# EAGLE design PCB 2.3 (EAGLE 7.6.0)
CNAME: DIY-Thermocam V2; CREVISION: 2.3; DESIGNER: Max Ritter
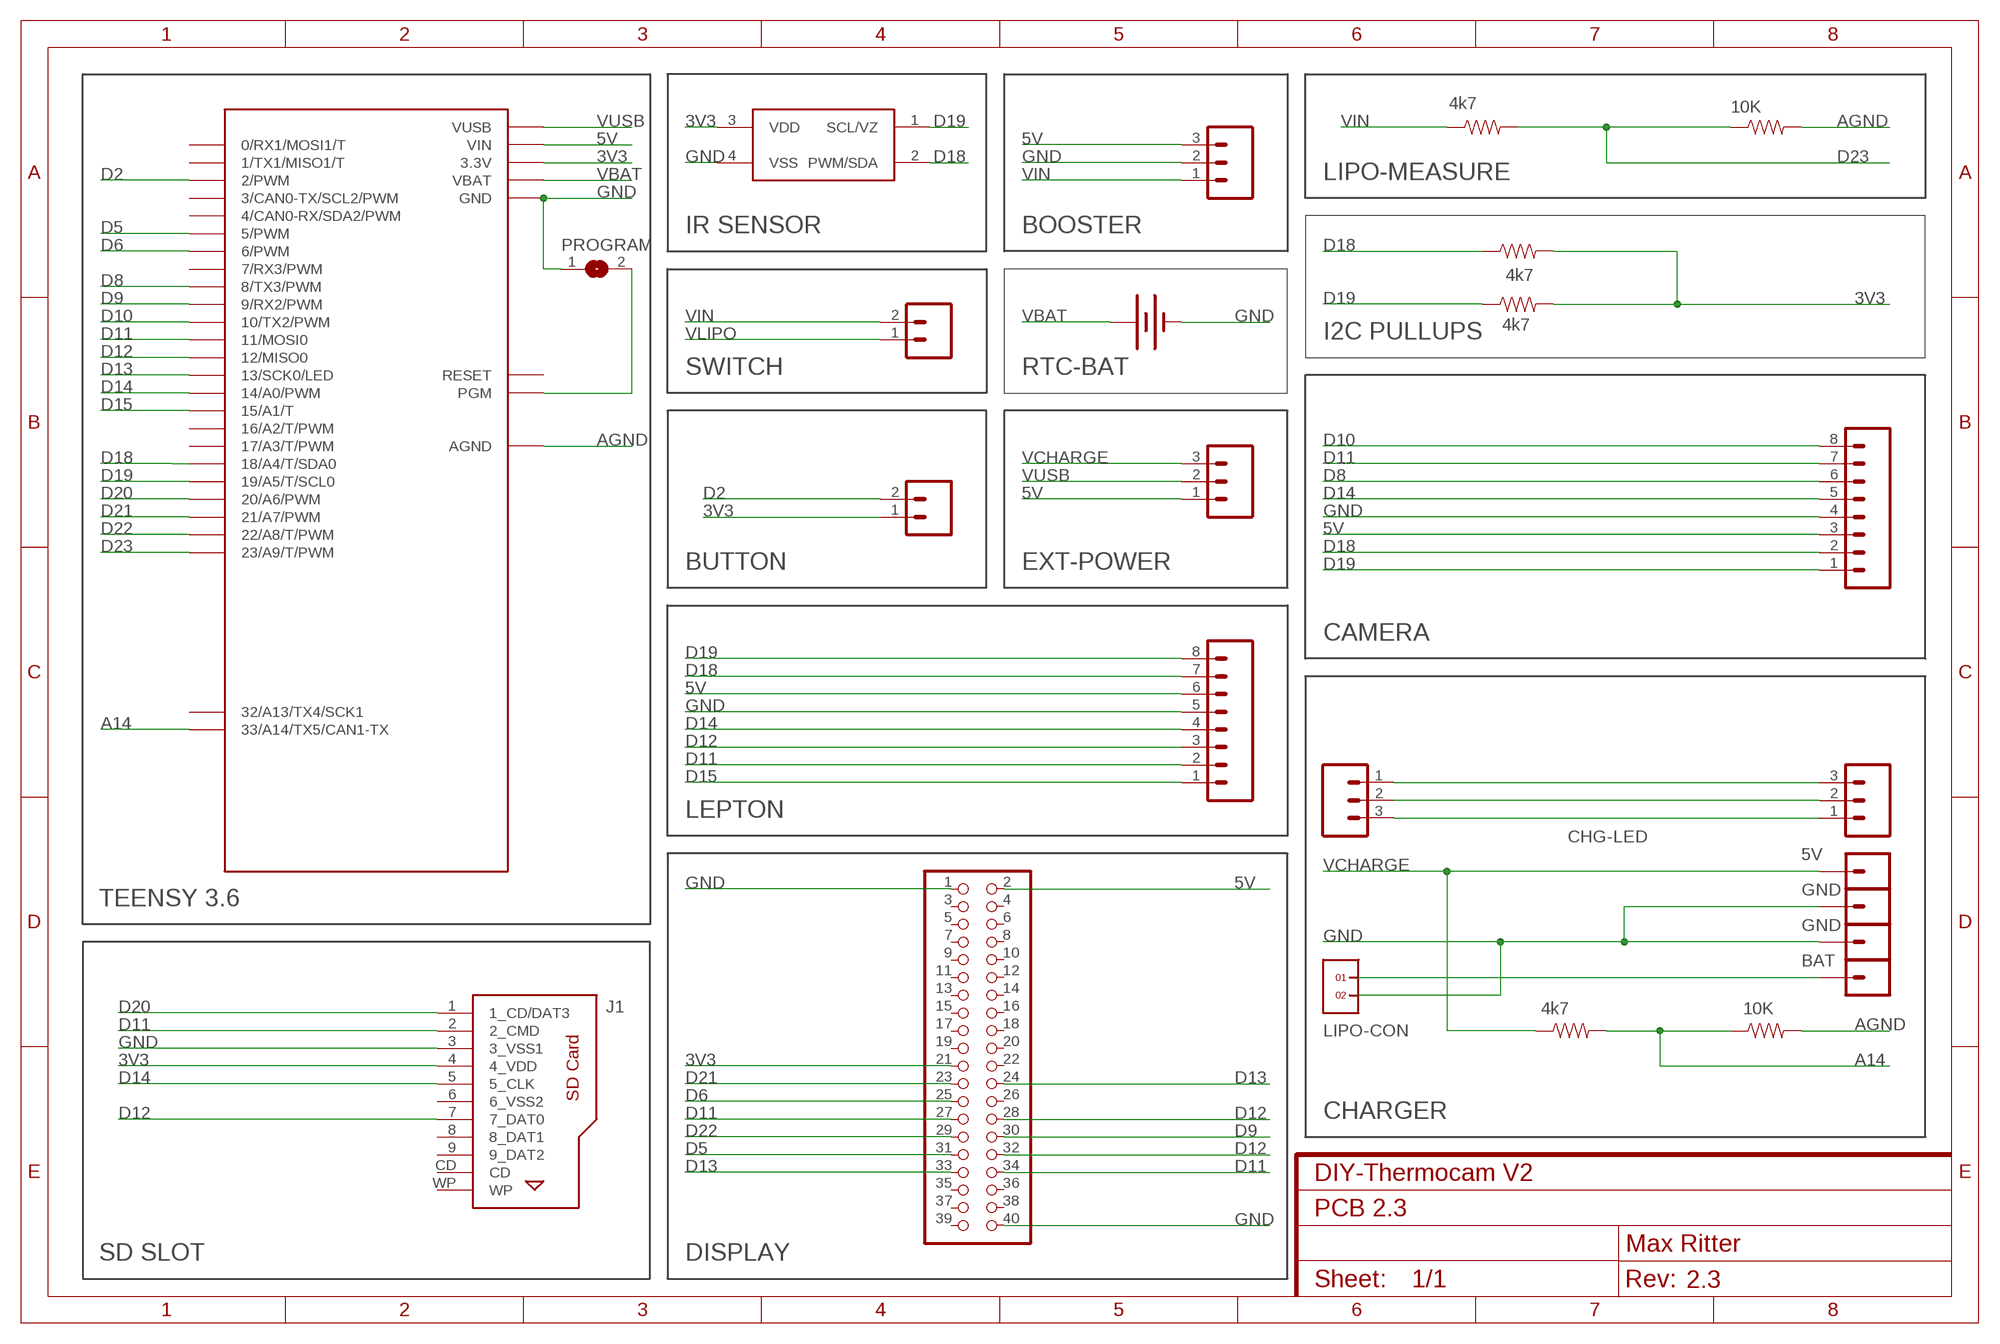
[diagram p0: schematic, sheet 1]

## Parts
BAT  BATTERY12PTH  [BATTCON_12MM_PTH]
BOOSTER  M03PTH  [1X03]
BUTTON  M02PTH  [1X02]
CHG-LED  M03PTH  [1X03]
EXT-POWER  M03PTH  [1X03]
J1  693063020911  [693063020911]
JP1  M01PTH  [1X01]
JP2  M01PTH  [1X01]
JP3  M01PTH  [1X01]
JP4  M01PTH  [1X01]
LASER1  M03PTH  [1X03]
LCD-HEADER  PINHD-2X20  [2X20]
LEPTON_MODULE  M08  [1X08_ROUND]
LEPTON_MODULE1  M08  [1X08_ROUND]
LIPO-CON  1X2  [1X2]
PROGRAM  SJ  [SJ]
R1  4k7  RESISTORPTH-1/4W  [AXIAL-0.4]
R2  10K  RESISTORPTH-1/4W  [AXIAL-0.4]
R3  4k7  RESISTORPTH-1/4W  [AXIAL-0.4]
R4  4k7  RESISTORPTH-1/4W  [AXIAL-0.4]
R5  10K  RESISTORPTH-1/4W  [AXIAL-0.4]
R6  4k7  RESISTORPTH-1/4W  [AXIAL-0.4]
SWITCH  M02PTH  [1X02]
U1  MLX90614_  [TO-39]
U$1  TEENSY_3.6_ALL_PINS  [TEENSY_3.6_ALL_PINS]

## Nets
3V3: BUTTON.1 J1.4(4_VDD) LCD-HEADER.21 R4.P$2 R6.P$2 U1.3(VDD) U$1.3.3V U$1.3.3V3(3.3V) U$1.3.3V4(3.3V)
5V: BOOSTER.3 EXT-POWER.1 LCD-HEADER.2 LEPTON_MODULE1.3 LEPTON_MODULE.6 U$1.VIN
A14: R3.P$2 R5.P$1 U$1.33/A14(33/A14/TX5/CAN1-TX)
AGND: R2.P$2 R5.P$2 U$1.AGND
D2: BUTTON.2 U$1.2(2/PWM)
D5: LCD-HEADER.31 U$1.5(5/PWM)
D6: LCD-HEADER.25 U$1.6(6/PWM)
D8: LEPTON_MODULE1.6 U$1.8(8/TX3/PWM)
D9: LCD-HEADER.30 U$1.9(9/RX2/PWM)
D10: LEPTON_MODULE1.8 U$1.10(10/TX2/PWM)
D11: J1.2(2_CMD) LCD-HEADER.27 LCD-HEADER.34 LEPTON_MODULE1.7 LEPTON_MODULE.2 U$1.11(11/MOSI0)
D12: J1.7(7_DAT0) LCD-HEADER.28 LCD-HEADER.32 LEPTON_MODULE.3 U$1.12(12/MISO0)
D13: LCD-HEADER.24 LCD-HEADER.33 U$1.13(13/SCK0/LED)
D14: J1.5(5_CLK) LEPTON_MODULE1.5 LEPTON_MODULE.4 U$1.14/A0(14/A0/PWM)
D15: LEPTON_MODULE.1 U$1.15/A1(15/A1/T)
D18: LEPTON_MODULE1.2 LEPTON_MODULE.7 R4.P$1 U1.2(PWM/SDA) U$1.18/A4(18/A4/T/SDA0)
D19: LEPTON_MODULE1.1 LEPTON_MODULE.8 R6.P$1 U1.1(SCL/VZ) U$1.19/A5(19/A5/T/SCL0)
D20: J1.1(1_CD/DAT3) U$1.20/A6(20/A6/PWM)
D21: LCD-HEADER.23 U$1.21/A7(21/A7/PWM)
D22: LCD-HEADER.29 U$1.22/A8(22/A8/T/PWM)
D23: R1.P$2 R2.P$1 U$1.23/A9(23/A9/T/PWM)
GND: BAT.GND(-) BOOSTER.2 J1.3(3_VSS1) JP1.1 JP2.1 LCD-HEADER.1 LCD-HEADER.40 LEPTON_MODULE1.4 LEPTON_MODULE.5 LIPO-CON.2 PROGRAM.1 U1.4(VSS) U$1.GND U$1.GND1(GND) U$1.GND6(GND)
N$4: CHG-LED.3 LASER1.1
N$16: CHG-LED.2 LASER1.2
N$18: CHG-LED.1 LASER1.3
N$42: PROGRAM.2 U$1.PGM
VBAT: BAT.VCC@1(+) U$1.VBAT
VCHARGE: EXT-POWER.3 JP4.1 R3.P$1
VIN: BOOSTER.1 R1.P$1 SWITCH.2
VLIPO: JP3.1 LIPO-CON.1 SWITCH.1
VUSB: EXT-POWER.2 U$1.VUSB
Unconnected: J1.6(6_VSS2) J1.8(8_DAT1) J1.9(9_DAT2) J1.CD J1.WP LCD-HEADER.3 LCD-HEADER.4 LCD-HEADER.5 LCD-HEADER.6 LCD-HEADER.7 LCD-HEADER.8 LCD-HEADER.9 LCD-HEADER.10 LCD-HEADER.11 LCD-HEADER.12 LCD-HEADER.13 LCD-HEADER.14 LCD-HEADER.15 LCD-HEADER.16 LCD-HEADER.17 LCD-HEADER.18 LCD-HEADER.19 LCD-HEADER.20 LCD-HEADER.22 LCD-HEADER.26 LCD-HEADER.35 LCD-HEADER.36 LCD-HEADER.37 LCD-HEADER.38 LCD-HEADER.39 U$1.0(0/RX1/MOSI1/T) U$1.1(1/TX1/MISO1/T) U$1.3(3/CAN0-TX/SCL2/PWM) U$1.4(4/CAN0-RX/SDA2/PWM) U$1.7(7/RX3/PWM) U$1.16/A2(16/A2/T/PWM) U$1.17/A3(17/A3/T/PWM) U$1.32/A13(32/A13/TX4/SCK1) U$1.RESET

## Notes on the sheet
- LIPO-MEASURE
- IR SENSOR | BOOSTER
- I2C PULLUPS
- SWITCH | RTC-BAT
- BUTTON | EXT-POWER
- CAMERA
- LEPTON
- 5V
- GND
- TEENSY 3.6
- GND
- BAT
- CHARGER
- SD SLOT | DISPLAY

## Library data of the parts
BAT = SparkFun-Electromechanical:BATTERY: Battery Holders
BOOSTER CHG-LED EXT-POWER LASER1 = SparkFun-Connectors:M03: Header 3 Standard 3-pin 0.1" header. Use with straight break away headers (SKU : PRT-00116), right angle break away headers (PRT-00553), swiss pins (PRT-00743), machine pins (PRT-00117), and female headers (PRT-00115). Molex polarized connector foot print use with SKU : PRT-08232 with associated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
BUTTON SWITCH = SparkFun-Connectors:M02: Standard 2-pin 0.1" header. Use with
J1 = EAGLE-INPUT_OUTPUT_CONNECTORS-rev16b:693063020911: WR-CRD SD CARD CONNECTOR PUSH & PULL SHORT TYPE WITH CARD DETECTION 9PINS=>Code : Con_I-O_COM_CRD_SD_Normal_693063020911 Details see: http://katalog.we-online.de/en/em/693_063_020_911 Created 2014-07-09, Karrer Zheng 2014 (C) Würth Elektronik
JP1-JP4 = SparkFun-Connectors:M01: Header 1
LCD-HEADER = pinhead:PINHD-2X20: PIN HEADER
LEPTON_MODULE LEPTON_MODULE1 = SparkFun-Connectors:M08: Header 8 Standard 8-pin 0.1" header. Use with straight break away headers (SKU : PRT-00116), right angle break away headers (PRT-00553), swiss pins (PRT-00743), machine pins (PRT-00117), and female headers (PRT-00115).
LIPO-CON = headers(2mm):1X2
PROGRAM = jumper:SJ: SMD solder JUMPER
R1-R6 = SparkFun-Resistors:RESISTOR: Resistor
U1 = SparkFun-Sensors:MLX90614: Non-contact PIR I2C interface temperature sensor
U$1 = Teensy_3_and_LC_Series_Boards_v1.4:TEENSY_3.6_ALL_PINS: All PIN version of the Teensy 3.6.

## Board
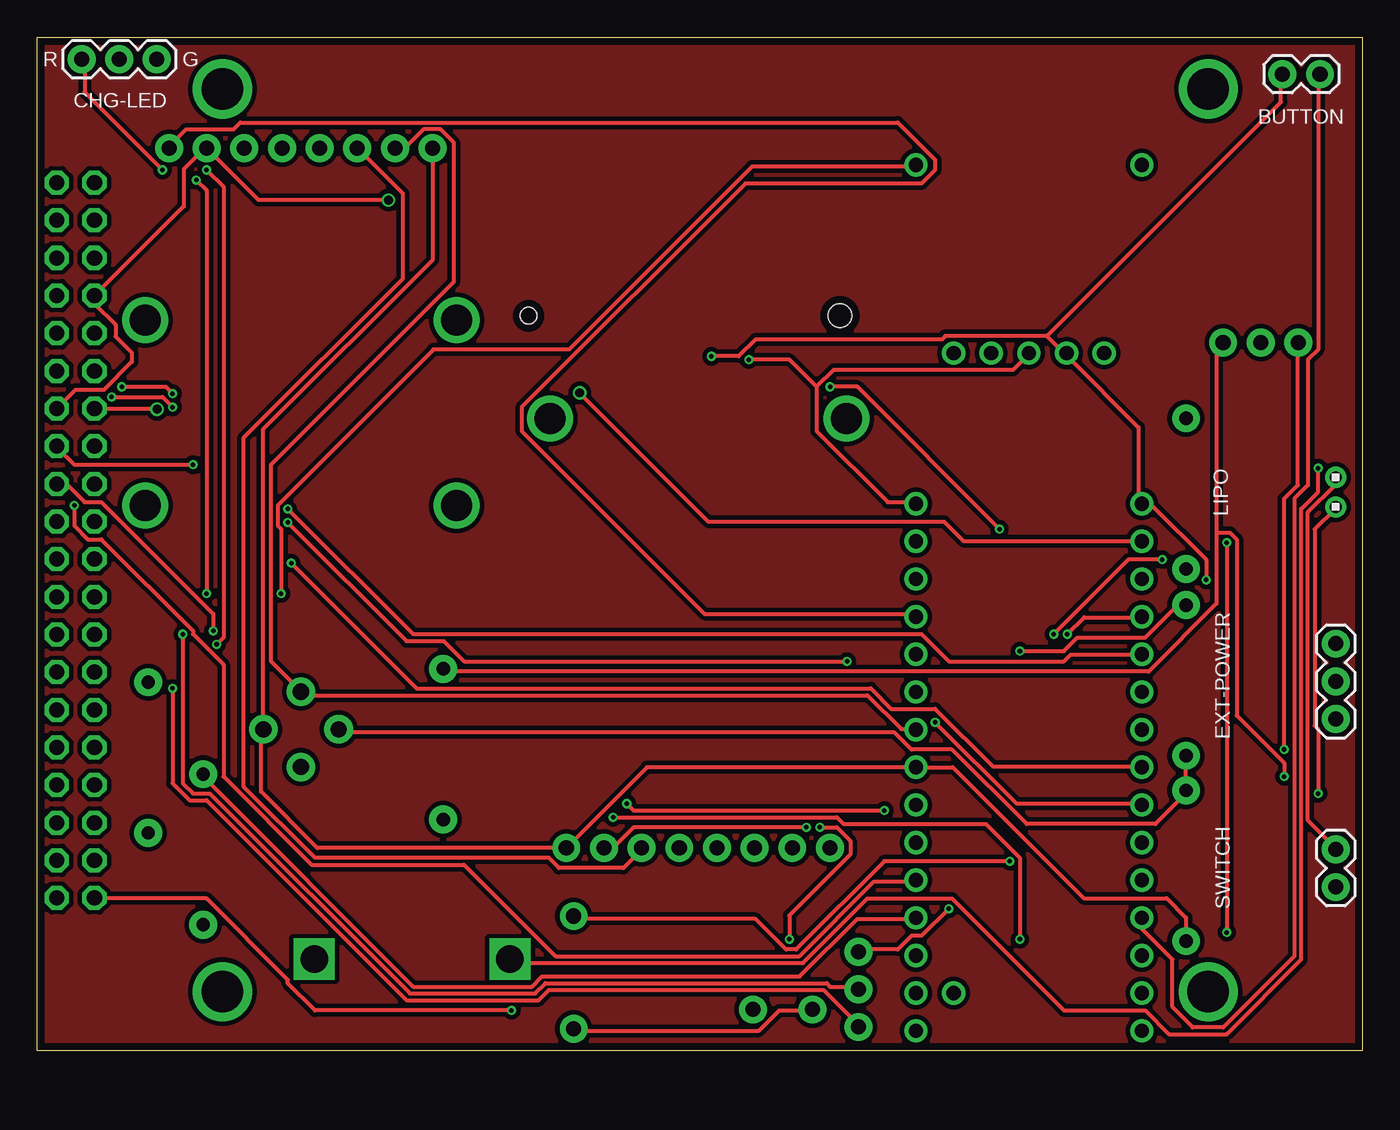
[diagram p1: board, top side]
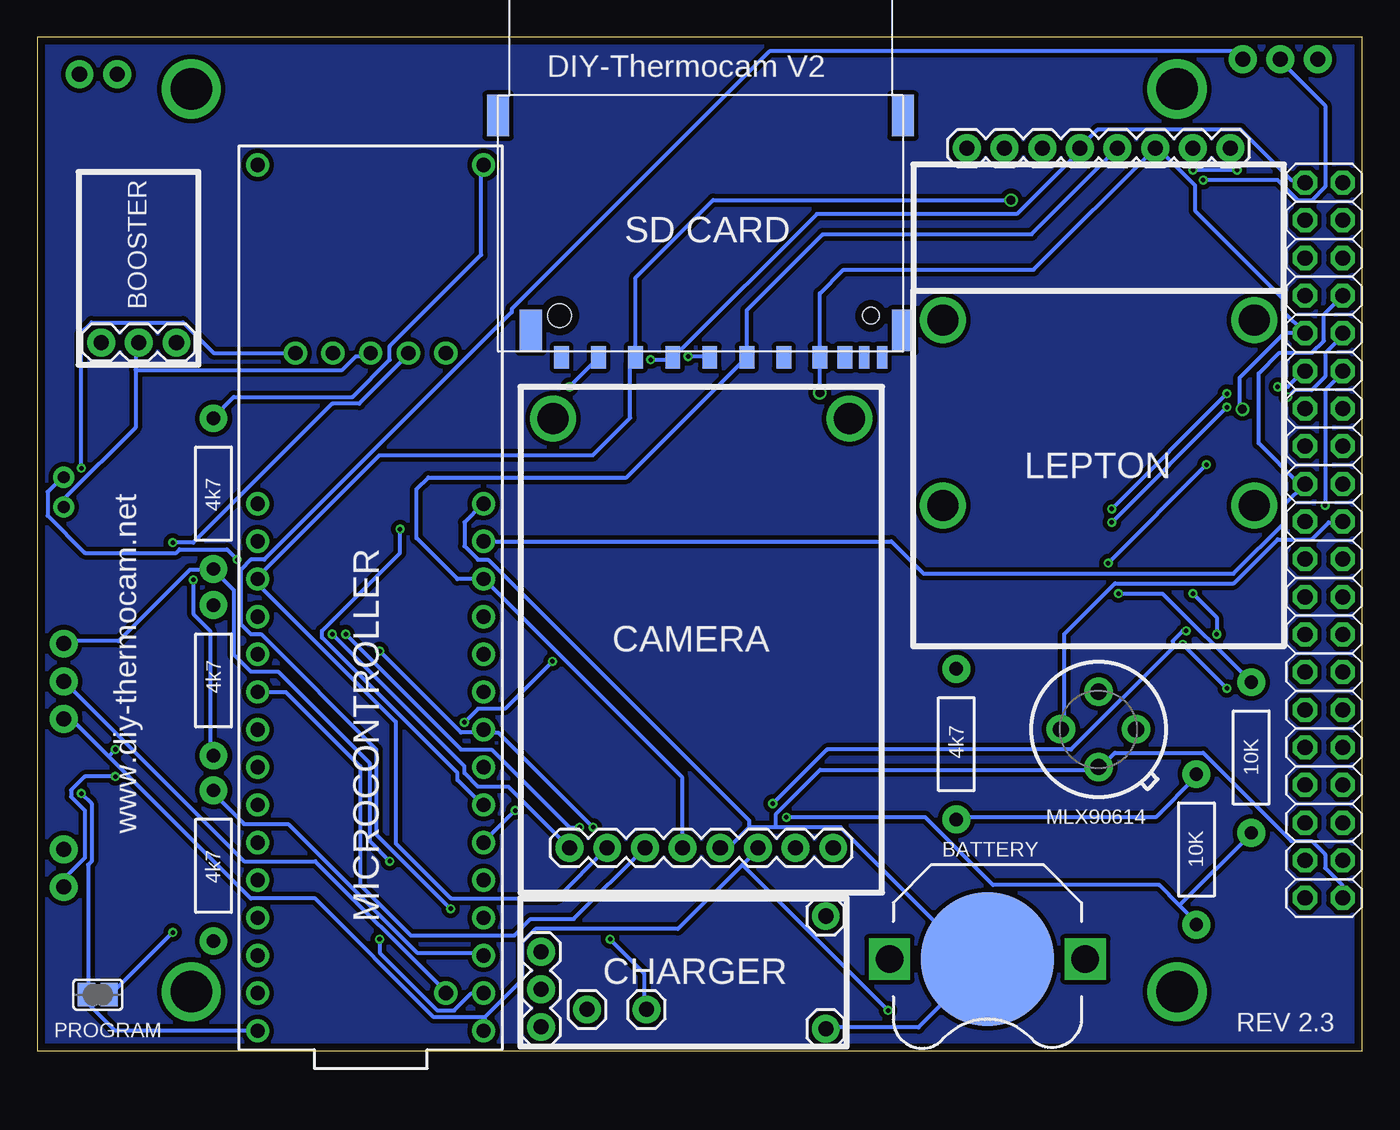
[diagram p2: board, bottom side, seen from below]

Size 89.4 x 68.4 mm. Coordinates in mm from the lower left corner, seen from the top.
Outline: 89.4,0 0,0 0,68.4 89.4,68.4 89.4,0
Copper layers (1*16): Top 0.035mm / dielectric 1.5mm / Bottom 0.035mm
Design rules "EagleRules *": minimum track width 10mil, minimum drill 12mil, track to track 8mil, track to pad 8mil, pad to pad 8mil, via to via 8mil, smd to smd 0mil, copper to edge 20mil, drill to drill 10mil, minimum pad ring 12mil, minimum via ring 6mil, stop-mask expansion 2mil, vias tented up to drill 25mil, thermal gap 10mil

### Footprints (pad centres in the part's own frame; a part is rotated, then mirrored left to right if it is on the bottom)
BATTCON_12MM_PTH = smd 9 x 9: GND 0,0 | drill 1.854 square: VCC@1 6.604,0; VCC@2 -6.604,0
1X03 = drill 1.016 pad 1.88: 1 0,0; 2 2.54,0; 3 5.08,0
1X02 = drill 1.016 pad 1.88: 1 0,0; 2 2.54,0
693063020911 = smd 1 x 1.5: 1 19.125,0; 2 16.625,0; 3 14.125,0; 4 11.625,0; 5 9.125,0; 6 6.625,0; 7 4.2,0; 8 2.5,0; 9 21.625,0 | smd 0.7 x 1.5: CD 1.2,0; WP 0,0 | smd 1.5 x 2.8: P$12 -1.4,-1.8; P$13 23.7,-1.8; P$14 -1.4,-16.3; P$15 25.9,-16.3 | hole 1.1: 0.75,-2.8 | hole 1.6: 21.75,-2.8
1X01 = drill 1.016 pad 1.88: 1 0,0
2X20 = drill 1.016 octagon: 1 -24.13,-1.27; 2 -24.13,1.27; 3 -21.59,-1.27; 4 -21.59,1.27; 5 -19.05,-1.27; 6 -19.05,1.27; 7 -16.51,-1.27; 8 -16.51,1.27; 9 -13.97,-1.27; 10 -13.97,1.27; 11 -11.43,-1.27; 12 -11.43,1.27; 13 -8.89,-1.27; 14 -8.89,1.27; 15 -6.35,-1.27; 16 -6.35,1.27; 17 -3.81,-1.27; 18 -3.81,1.27; 19 -1.27,-1.27; 20 -1.27,1.27; 21 1.27,-1.27; 22 1.27,1.27; 23 3.81,-1.27; 24 3.81,1.27; 25 6.35,-1.27; 26 6.35,1.27; 27 8.89,-1.27; 28 8.89,1.27; 29 11.43,-1.27; 30 11.43,1.27; 31 13.97,-1.27; 32 13.97,1.27; 33 16.51,-1.27; 34 16.51,1.27; 35 19.05,-1.27; 36 19.05,1.27; 37 21.59,-1.27; 38 21.59,1.27; 39 24.13,-1.27; 40 24.13,1.27
1X08_ROUND = drill 1.016 pad 1.88: 1 0,0; 2 2.54,0; 3 5.08,0; 4 7.62,0; 5 10.16,0; 6 12.7,0; 7 15.24,0; 8 17.78,0
1X2 = drill 0.8 pad 1.422: 1 -1,0; 2 1,0
SJ = smd 1.168 x 1.6: 1 -0.762,0; 2 0.762,0
AXIAL-0.4 = drill 0.9 pad 1.88: P$1 -5.08,0; P$2 5.08,0
TO-39 = drill 1.1 pad 1.93: 1 2.54,0; 2 0,2.54; 3 -2.54,0; 4 0,-2.54
TEENSY_3.6_ALL_PINS = drill 0.965: 0 -7.62,25.4; 1 -7.62,22.86; 2 -7.62,20.32; 3 -7.62,17.78; 3.3V 7.62,22.86; 3.3V3 -7.62,-7.62; 3.3V4 -2.54,-17.78; 4 -7.62,15.24; 5 -7.62,12.7; 6 -7.62,10.16; 7 -7.62,7.62; 8 -7.62,5.08; 9 -7.62,2.54; 10 -7.62,0; 11 -7.62,-2.54; 12 -7.62,-5.08; 13 7.62,-5.08; 14/A0 7.62,-2.54; 15/A1 7.62,0; 16/A2 7.62,2.54; 17/A3 7.62,5.08; 18/A4 7.62,7.62; 19/A5 7.62,10.16; 20/A6 7.62,12.7; 21/A7 7.62,15.24; 22/A8 7.62,17.78; 23/A9 7.62,20.32; 32/A13 -7.62,-30.48; 33/A14 7.62,-30.48; AGND 7.62,25.4; GND -7.62,27.94; GND1 7.62,-7.62; GND6 0,-17.78; PGM 2.54,-17.78; RESET 5.08,-17.78; VBAT -5.08,-17.78; VIN 7.62,27.94; VUSB 5.08,25.4

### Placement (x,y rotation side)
BAT  25.3,6.2 180 bottom
BOOSTER  80,47.8 180 bottom
BUTTON  84,65.9 0 top
CHG-LED  3,66.9 0 top
EXT-POWER  87.6,22.4 90 top
J1  32.4,46.8 180 bottom
JP1  36.2,1.5 0 bottom
JP2  52.3,2.8 0 bottom
JP3  48.3,2.8 0 bottom
JP4  36.2,9.1 0 bottom
LASER1  55.4,6.7 270 bottom
LCD-HEADER  2.6,34.45 90 bottom
LEPTON_MODULE  8.9,60.9 180 bottom
LEPTON_MODULE1  35.7,13.7 180 bottom
LIPO-CON  87.6,37.7 270 top
PROGRAM  85.3,3.8 0 bottom
R1  27.4,20.7 270 bottom
R2  11.2,13.6 270 bottom
R3  77.5,37.6 90 bottom
R4  77.5,25 270 bottom
R5  7.5,19.8 270 bottom
R6  77.5,12.5 90 bottom
SWITCH  87.6,13.6 270 top
U1  17.8,21.7 0 bottom
U$1  66.9,29.3 180 top

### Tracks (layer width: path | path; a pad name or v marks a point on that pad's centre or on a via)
3V3  (via drill 0.3)
  Top 0.254: R4.P$2 77.5,19.89 77.5,17.6 R6.P$2 77.5,17.37 75.44,15.32 66.75,15.32 61.72,20.34 58.98,20.34 57.84,21.49 20.34,21.49 U1.3 | v45.49,46.86 47.32,46.86 48.46,48.01 61.04,48.01 61.27,48.23 68.12,48.23 | 68.12,48.23 69.27,47.09 U$1.3.3V4 69.49,46.86 74.3,42.06 74.3,37.03 U$1.3.3V3 74.52,36.8 75.21,36.8 78.87,33.15 v78.87,31.77 | 68.12,48.23 83.9,64.01 83.9,65.84 BUTTON.1
  Bottom 0.254: LCD-HEADER.21 1.37,35.66 2.29,35.66 3.43,34.52 5.71,34.52 8.69,31.55 16.69,31.55 20.12,28.12 20.12,21.72 U1.3 | U$1.3.3V 59.44,6.63 63.78,6.63 72.47,15.32 75.44,15.32 77.5,17.37 R6.P$2 | v45.49,46.86 44.12,46.86 J1.4 | v78.87,31.77 78.87,29.49 77.72,28.35 77.72,20.12 R4.P$2
5V  (via drill 0.3)
  Top 0.254: v32,2.74 18.75,2.74 16.92,4.57 16.92,4.8 11.43,10.29 3.89,10.29 LCD-HEADER.2 | LEPTON_MODULE.6 21.72,60.81 24.69,57.84 24.69,52.12 13.95,41.38 13.95,17.83 18.75,13.03 34.52,13.03 35.2,12.34 39.55,12.34 40.69,13.49 LEPTON_MODULE1.3 | v84.12,20.34 84.12,37.26 85.04,38.18 85.04,47.78 BOOSTER.3
  Bottom 0.254: 59.21,2.29 59.21,1.37 U$1.VIN | 59.21,2.29 56.69,4.8 56.69,7.32 55.78,8.23 46.18,8.23 41.83,12.57 | 41.83,12.57 40.92,13.49 LEPTON_MODULE1.3 | 41.83,12.57 v32,2.74 | 84.58,19.89 74.98,10.29 70.64,10.29 62.64,2.29 59.21,2.29 | 84.58,19.89 86.87,22.17 87.55,22.17 EXT-POWER.1 | 84.58,19.89 v84.12,20.34
A14  (via drill 0.3)
  Top 0.254: v16.46,30.86 16.46,35.2 16.23,35.43 16.23,36.8 26.75,47.32 35.89,47.32 48.23,59.66 59.21,59.66 U$1.33/A14
  Bottom 0.254: U$1.33/A14 59.44,59.66 59.44,53.72 65.61,47.55 65.61,46.63 68.12,44.12 76.12,44.12 77.5,42.75 R3.P$2 | v16.46,30.86 13.49,30.86 7.54,24.92 R5.P$1
AGND  (via drill 0.3)
  Top 0.254: v66.29,7.54 66.29,13.03 64.01,15.32 54.41,15.32 53.95,15.77 v38.86,15.77
  Bottom 0.254: v66.29,7.54 66.29,6.63 62.41,2.74 61.27,2.74 60.12,3.89 59.44,3.89 U$1.AGND | v38.86,15.77 29.49,15.77 24.92,11.2 13.72,11.2 12.34,9.83 | 12.34,9.83 11.2,8.69 R2.P$2 | 12.34,9.83 7.54,14.63 R5.P$2
D2
  Top 0.254: U$1.2 74.52,8.91 74.52,8.23 76.58,6.17 76.58,2.97 77.95,1.6 80.01,1.6 84.81,6.4 84.81,37.26 85.72,38.18 85.72,46.63 86.41,47.32 86.41,65.84 BUTTON.2
D5  (via drill 0.3)
  Top 0.254: v60.58,22.17 66.06,16.69 74.3,16.69 U$1.5 | v54.63,26.29 28.8,26.29 27.43,27.66 24.92,27.66 v16.92,35.66 | v9.14,43.43 8.46,44.12 v5.03,44.12
  Bottom 0.254: v60.58,22.17 59.66,23.09 57.84,23.09 v54.63,26.29 | v9.14,43.43 v16.92,35.66 | v5.03,44.12 4.57,44.58 3.43,44.58 2.52,45.49 2.52,47.09 1.37,48.23 LCD-HEADER.31
D6  (via drill 0.3)
  Top 0.254: v17.14,32.92 25.6,24.46 56.24,24.46 57.61,23.09 60.58,23.09 64.47,19.2 74.3,19.2 U$1.6 | v10.52,39.55 2.52,39.55 1.37,40.69 LCD-HEADER.25
  Bottom 0.254: v10.52,39.55 v17.14,32.92
D8
  Bottom 0.254: U$1.8 72.62,24.22 67.6,19.2 67.6,11.2 64.2,7.8 57.2,7.8 56.1,8.9 53.2,8.9 LEPTON_MODULE1.6
D9  (via drill 0.3)
  Top 0.254: v16.92,36.58 25.38,28.12 59.66,28.12 61.49,26.29 69.27,26.29 69.72,26.75 74.3,26.75 U$1.9 | v9.14,44.35 8.69,44.81 v5.71,44.81
  Bottom 0.254: v9.14,44.35 v16.92,36.58 | v5.71,44.81 5.03,44.81 3.89,45.95 LCD-HEADER.30
D10  (via drill 0.3)
  Top 0.254: v69.49,28.12 70.64,29.26 74.3,29.26 U$1.10
  Bottom 0.254: v69.49,28.12 60.58,19.2 60.58,18.75 59.66,17.83 57.61,17.83 53.49,13.72 LEPTON_MODULE1.8
D11  (via drill 0.6)
  Top 0.254: v23.7,57.4 14.94,57.4 LEPTON_MODULE.2 11.3,60.9 9.9,59.5 9.9,56.99 LCD-HEADER.34 3.87,50.43 5.3,49 5.3,48.2 6.4,47.1 6.4,46.5 4.5,44.6 2.59,44.6 LCD-HEADER.27
  Bottom 0.254: LEPTON_MODULE1.7 54.34,10.3 61.5,10.3 65.2,14 65.2,22.2 74.52,31.52 U$1.11 74.52,31.98 66.3,40.2 51.9,40.2 49.4,42.7 49.4,46.42 J1.2 49.02,52.17 43.8,57.4 v23.7,57.4
D12  (via drill 0.6)
  Top 0.254: U$1.12 62.52,34.38 61.2,35.7 45.3,35.7 v36.6,44.4 | v8.1,43.3 3.91,43.3 LCD-HEADER.28
  Bottom 0.254: v36.6,44.4 J1.7 36.6,51.1 35,52.7 22.18,52.7 LEPTON_MODULE.3 13.8,60.9 11.3,58.4 11.3,56.7 5.4,50.8 5.4,49.95 LCD-HEADER.32 5.28,48.42 8.3,45.4 8.3,43.5 v8.1,43.3
D13
  Bottom 0.254: U$1.13 31.78,34.38 29.6,32.2 8.7,32.2 5.2,35.7 5.2,36.93 LCD-HEADER.24 4.26,38.26 7,41 7,45.7 5.6,47.1 3.4,47.1 2.6,47.9 2.6,49.69 LCD-HEADER.33
D14
  Bottom 0.254: LEPTON_MODULE1.5 45.9,13.74 45.9,18.5 59.24,31.84 U$1.14/A0 61.04,31.84 63.8,34.6 63.8,37.9 63,38.7 49.62,38.7 J1.5 41.52,49.98 36.4,55.1 22.32,55.1 LEPTON_MODULE.4
D15
  Top 0.254: U$1.15/A1 59.21,29.49 45.03,29.49 32.69,41.83 32.69,43.43 47.78,58.52 59.66,58.52 60.58,59.44 60.58,60.12 58.06,62.64 13.72,62.64 13.26,62.18 10.06,62.18 8.91,61.04 LEPTON_MODULE.1
D18  (via drill 0.3)
  Top 0.254: U$1.18/A4 59.21,21.72 58.29,21.72 56.01,24 18.06,24 17.83,24.23 U1.2 17.6,24.46 15.77,26.29 15.77,39.55 28.12,51.89 28.12,61.27 27.2,62.18 26.06,62.18 24.92,61.04 24.23,61.04 LEPTON_MODULE.7 | v51.89,15.09 40.23,15.09 38.86,13.72 38.41,13.72 LEPTON_MODULE1.2 | v66.29,26.98 69.27,26.98 70.18,27.89 74.75,27.89 76.81,29.95 77.5,29.95 R4.P$1
  Bottom 0.254: v51.89,15.09 58.29,21.49 59.21,21.49 U$1.18/A4 59.44,21.49 60.81,21.49 v66.29,26.98
D19
  Top 0.254: R6.P$1 77.5,9 76.2,10.3 70.6,10.3 61.76,19.14 U$1.19/A5 41.14,19.14 LEPTON_MODULE1.1 18.9,13.7 15.1,17.5 15.1,21.54 U1.1 15.26,41.96 26.7,53.4 26.7,60.88 LEPTON_MODULE.8
D20  (via drill 0.3)
  Top 0.254: v53.49,44.81 55.32,44.81 v64.92,35.2
  Bottom 0.254: v53.49,44.81 51.66,46.63 J1.1 | v64.92,35.2 64.92,33.6 70.18,28.35 70.18,27.89 61.04,18.75 61.04,18.29 59.44,16.69 U$1.20/A6
D21  (via drill 0.3)
  Top 0.254: v57.15,16.23 40.23,16.23 v39.78,16.69 | v11.89,28.35 11.89,29.49 4.34,37.03 3.2,37.03 2.06,38.18 1.37,38.18 LCD-HEADER.23
  Bottom 0.254: v57.15,16.23 59.21,14.17 U$1.21/A7 | v39.78,16.69 36.12,20.34 19.66,20.34 12.8,27.2 12.8,27.66 12.12,28.35 v11.89,28.35
D22  (via drill 0.3)
  Top 0.254: v2.52,36.8 2.52,35.43 3.43,34.52 4.34,34.52 10.52,28.35 10.52,28.12 12.57,26.06 12.57,18.52 18.52,12.57 28.8,12.57 34.98,6.4 51.44,6.4 56.46,11.43 59.21,11.43 U$1.22/A8
  Bottom 0.254: v2.52,36.8 2.52,44.58 1.37,45.72 LCD-HEADER.29
D23
  Top 0.254: U$1.23/A9 59.21,8.91 55.32,8.91 51.44,5.03 34.06,5.03 33.38,4.34 25.38,4.34 11.2,18.52 R2.P$1
  Bottom 0.254: R1.P$2 27.2,15.77 13.95,15.77 11.2,18.52 R2.P$1
GND  (via drill 0.3)
  Top 0.254: JP2.1 52.12,2.74 50.06,2.74 48.69,1.37 36.35,1.37 JP1.1 | 52.58,44.81 52.58,41.83 57.38,37.03 59.21,37.03 U$1.GND1 | 52.58,44.81 53.72,45.95 65.84,45.95 66.75,46.86 U$1.GND6 | v86.41,17.37 86.41,21.72 86.18,21.95 86.18,35.2 87.55,36.58 LIPO-CON.2 | v48.01,46.63 50.75,46.63 52.58,44.81
  Bottom 0.254: LCD-HEADER.1 1.37,10.52 1.37,11.2 2.52,12.34 2.52,13.26 3.43,14.17 4.8,14.17 10.74,20.12 16.69,20.12 17.6,19.2 U1.4 17.83,18.97 36.58,18.97 39.55,16 39.55,15.09 | 25.83,5.71 25.38,6.17 BAT.GND 25.83,5.71 | 25.83,5.71 29.95,1.6 36.12,1.6 JP1.1 | 41.38,15.09 42.75,13.72 43.2,13.72 LEPTON_MODULE1.4 | 39.55,15.09 35.2,15.09 25.83,5.71 | 39.55,15.09 41.38,15.09 | LCD-HEADER.40 3.89,58.75 4.8,58.75 8.23,62.18 17.83,62.18 18.97,61.04 LEPTON_MODULE.5 18.97,60.81 23.32,56.46 36.8,56.46 46.41,46.86 J1.3 46.63,46.63 v48.01,46.63 | U$1.GND 74.52,1.37 84.12,1.37 85.95,3.2 85.95,3.66 PROGRAM.1 85.95,3.89 85.95,12.57 85.72,12.8 85.72,16.69 v86.41,17.37 | 82.75,45.95 82.75,47.78 BOOSTER.2 | 82.75,45.95 82.75,42.06 87.55,37.26 87.55,36.8 LIPO-CON.2 | 82.75,45.95 68.81,45.95 67.89,46.86 66.98,46.86 U$1.GND6 | 41.38,15.09 41.38,15.54 58.98,33.15 59.66,33.15 60.58,34.06 60.58,35.66 59.44,36.8 U$1.GND1
N$1  (via drill 2.8 pad 4)
  other vias: 12.5,64.9
N$2
  pour Top (isolate 0.305): 0,0 89.4,0 89.4,68.4 0,68.4
N$3
  pour Bottom (isolate 0.305): 0,0 89.4,0 89.4,68.4 0,68.4
N$4  (via drill 0.3)
  Top 0.254: v61.49,9.6 59.66,7.77 58.98,7.77 58.06,6.86 55.55,6.86 LASER1.1
  Bottom 0.254: v61.49,9.6 66.52,14.63 66.52,20.34 74.3,28.12 74.98,28.12 75.67,28.8 75.67,32.46 74.98,33.15 74.07,33.15 57.38,49.84 57.38,50.06 40.01,67.44 8.69,67.44 8.23,66.98 CHG-LED.3
N$6  (via drill 2.1 pad 3.12)
  other vias: 28.3,36.8
N$7  (via drill 2.8 pad 4)
  other vias: 12.5,4
N$8  (via drill 2.1 pad 3.12)
  other vias: 34.6,42.67
N$9  (via drill 2.1 pad 3.12)
  other vias: 54.6,42.67
N$10  (via drill 2.8 pad 4)
  other vias: 79,4
N$11  (via drill 2.8 pad 4)
  other vias: 79,64.9
N$12  (via drill 2.1 pad 3.12)
  other vias: 7.3,49.3
N$13  (via drill 2.1 pad 3.12)
  other vias: 7.3,36.8
N$14  (via drill 2.1 pad 3.12)
  other vias: 28.3,49.3
N$16  (via drill 0.3)
  Top 0.254: v9.83,28.12 9.83,18.06 10.52,17.37 11.66,17.37 25.15,3.89 33.6,3.89 34.29,4.57 53.26,4.57 53.49,4.34 55.32,4.34 LASER1.2 | v11.43,30.86 11.43,58.06 v10.74,58.75
  Bottom 0.254: v9.83,28.12 9.83,29.26 v11.43,30.86 | v10.74,58.75 5.71,58.75 4.34,57.38 3.43,57.38 2.52,58.29 2.52,63.78 5.49,66.75 CHG-LED.2
N$18  (via drill 0.3)
  Top 0.254: v9.14,24.46 9.14,18.06 10.29,16.92 11.43,16.92 24.92,3.43 33.83,3.43 34.52,4.12 53.03,4.12 55.32,1.83 LASER1.3 | v12.12,27.43 12.57,27.89 12.57,58.29 v11.43,59.44 | v8.46,59.44 3.2,64.69 3.2,66.75 CHG-LED.1
  Bottom 0.254: v12.12,27.43 v9.14,24.46 | v8.46,59.44 v11.43,59.44
N$42  (via drill 0.3)
  Top 0.254: v80.24,34.29 v80.24,8
  Bottom 0.254: v80.24,8 84.35,3.89 PROGRAM.2 | v80.24,34.29 78.87,34.29 69.49,43.66 67.67,43.66 64.47,46.86 U$1.PGM
VBAT  (via drill 0.3)
  Top 0.254: v86.41,39.32 86.41,37.72 85.27,36.58 85.27,6.17 80.24,1.14 76.35,1.14 74.75,2.74 69.27,2.74 61.72,10.29 56.01,10.29 51.66,5.94 32.23,5.94 32,6.17 BAT.VCC@1
  Bottom 0.254: v86.41,39.32 86.41,48.46 85.72,49.15 79.55,49.15 77.5,47.09 72.01,47.09 U$1.VBAT
VCHARGE  (via drill 0.3)
  Top 0.254: v65.61,12.8 57.15,12.8 51.21,6.86 50.52,6.86 48.46,8.91 36.35,8.91 JP4.1
  Bottom 0.254: v65.61,12.8 66.98,14.17 66.98,19.43 73.15,25.6 74.98,25.6 76.12,26.75 76.12,31.09 77.5,32.46 R3.P$1 77.72,32.46 79.1,32.46 83.9,27.66 87.55,27.66 EXT-POWER.3
VIN  (via drill 0.3)
  Top 0.254: 79.55,34.98 79.55,47.55 79.78,47.78 BOOSTER.1 | 79.55,34.98 79.55,30.18 74.98,25.6 27.43,25.6 R1.P$1 | v84.12,18.52 84.12,19.43 80.92,22.63 80.92,34.52 80.47,34.98 79.55,34.98
  Bottom 0.254: v84.12,18.52 86.18,18.52 87.1,17.6 87.1,17.14 86.18,16.23 86.18,13.03 87.55,11.66 87.55,11.2 SWITCH.2
VLIPO  (via drill 0.3)
  Top 0.254: LIPO-CON.1 87.55,38.63 87.55,38.18 85.72,36.35 85.72,15.54 87.55,13.72 SWITCH.1 | v50.75,7.54 50.75,9.14 54.86,13.26 54.86,14.17 53.95,15.09 v52.81,15.09 | v68.58,28.12 73.61,33.15 v75.89,33.15
  Bottom 0.254: v50.75,7.54 48.46,5.26 48.46,2.97 JP3.1 | v52.81,15.09 53.49,15.09 58.75,20.34 60.81,20.34 v68.58,28.12 | v75.89,33.15 76.58,33.83 79.78,33.83 80.01,33.6 86.18,33.6 88.7,36.12 88.7,37.72 87.78,38.63 LIPO-CON.1
VUSB
  Bottom 0.254: U$1.VUSB 61.95,4.12 70.64,12.8 75.44,12.8 87.55,24.92 EXT-POWER.2

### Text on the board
tPlace: R | G | LIPO
bPlace: DIY-Thermocam V2 | SD CARD | BOOSTER | LEPTON | www.diy-thermocam.net | MICROCONTROLLER | CAMERA | MLX90614 | BATTERY | CHARGER | REV 2.3 | PROGRAM

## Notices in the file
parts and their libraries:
SparkFun-Aesthetics: Licensing: Creative Commons ShareAlike 4.0 International - https://creativecommons.org/licenses/by-sa/4.0
EAGLE-INPUT_OUTPUT_CONNECTORS-rev16b: Copyright: Würth Elektronik
